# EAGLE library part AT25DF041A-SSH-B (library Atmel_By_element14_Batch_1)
Serial Flash Memory
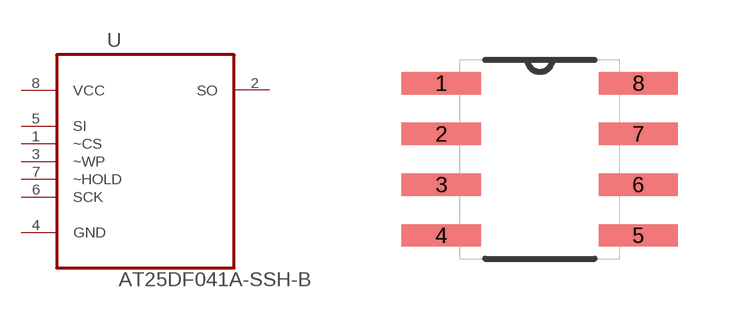
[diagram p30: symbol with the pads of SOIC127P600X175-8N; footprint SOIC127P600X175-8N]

Designator prefix U

## AT25DF041A-SSH-B (MPN: AT25DF041A-SSH-B; OC_FARNELL: 1715441; OC_NEWARK: 15R0306; PACKAGE: SOIC-8; SUPPLIER: Atmel)  [SOIC127P600X175-8N]
1  ~CS  in
2  SO  out
3  ~WP  in
4  GND  pas
5  SI  in
6  SCK  in
7  ~HOLD  in
8  VCC  pwr

## Footprint SOIC127P600X175-8N (pad centres in mm)
smd 1.981 x 0.559: 1 -2.464,1.905; 2 -2.464,0.635; 3 -2.464,-0.635; 4 -2.464,-1.905; 5 2.464,-1.905; 6 2.464,-0.635; 7 2.464,0.635; 8 2.464,1.905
